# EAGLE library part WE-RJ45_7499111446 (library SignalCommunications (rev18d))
Order Code 7499111446 Design THT xBase-T 10/100/1000 Base-T Ports 1x1 Application Standard Tab Position DOWN LED (Left-Right) GREEN/YELLOW-GREEN/YELLOW EMI Fingers yes Details see: http://katalog.we-online.de/en/pbs/WE-LAN_RJ45/7499111446? Updated by Yingchun Shan 2016-08-29 2016(C) Würth Elektronik
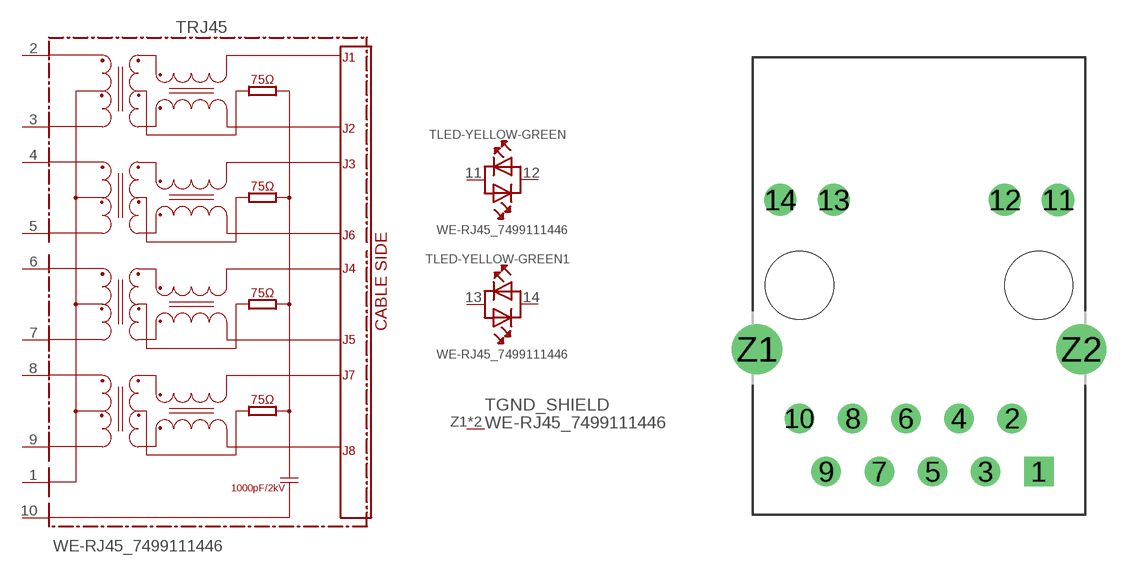
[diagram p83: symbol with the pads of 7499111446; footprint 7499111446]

Designator prefix T; gates RJ45=7499111446 LED-YELLOW-GREEN=LED-DUAL-1 LED-YELLOW-GREEN1=LED-DUAL-1 GND_SHIELD=GND_PIN

## WE-RJ45_7499111446 (COMPANY-URL: http://www.we-online.de; CREATED-BY: Christin Zierenner; CREATED-DATE: AUG 2012; DATASHEET-URL: http://katalog.we-online.de/kataloge/eisos/media/pdf/7499111446.pdf; MANUFACTURER: Würth Elektronik eiSos GmbH)  [7499111446]
1  RJ45:1
2  RJ45:2
3  RJ45:3
4  RJ45:4
5  RJ45:5
6  RJ45:6
7  RJ45:7
8  RJ45:8
9  RJ45:9
10  RJ45:10  pwr
11  LED-YELLOW-GREEN:AK1  pas
12  LED-YELLOW-GREEN:AK2  pas
13  LED-YELLOW-GREEN1:AK1  pas
14  LED-YELLOW-GREEN1:AK2  pas
Z1  GND_SHIELD:1  pwr
Z2  GND_SHIELD:1  pwr

## Footprint 7499111446 (pad centres in mm)
MAX HEIGHT=13.95mm PORTS----1X1 LED --YES
drill 0.9 square: 1 5.715,-8.89
drill 0.9: 2 4.445,-6.35; 3 3.175,-8.89; 4 1.905,-6.35; 5 0.635,-8.89; 6 -0.635,-6.35; 7 -1.905,-8.89; 8 -3.175,-6.35; 9 -4.445,-8.89; 10 -5.715,-6.35
drill 1.025: 11 6.63,4.08
drill 1.02: 12 4.09,4.08; 13 -4.09,4.08; 14 -6.63,4.08
drill 1.6: Z1 -7.745,-3.05; Z2 7.745,-3.05
hole 3.25 at 5.715,0
hole 3.25 at -5.715,0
